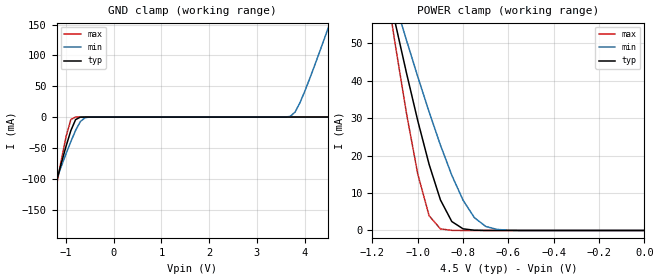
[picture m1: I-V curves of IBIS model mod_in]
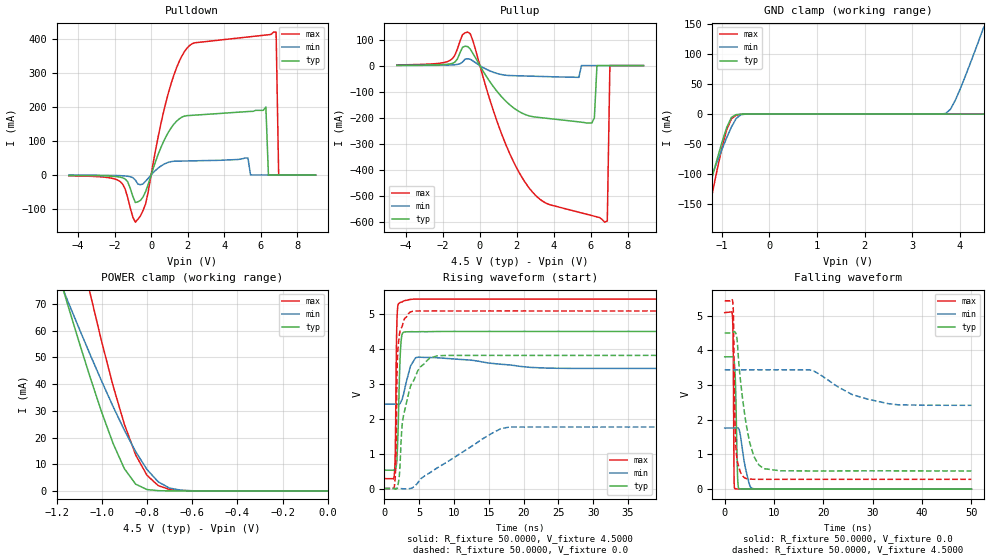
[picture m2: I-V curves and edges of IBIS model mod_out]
| IBIS file 54ac16244.ibs created by s2ibis3 verion 1.1
| North Carolina State University, ERL, 2006
[IBIS ver]  4.0
[File name] 54ac16244_4v5_rev1.ibs
[File Rev] 1.0
[Date]   19 Oct 2011
[Source] CAD & Design Solution (Catania) - STMicroelectronics
[Notes]
  (Note1) This IBIS model is the model of the product with package
   (Flat48 package elements);
  (Note2) This IBIS model is extracted with nominal 4.5V power supply
   (min:3.0V, typ:4.5V, max:5.5V);
  (Note3) This model has few Warnings about the non-monotonicity
   of I-V curves, but they are not indicative of problems
   inside the model;
[Copyright] (c) 2011 STMicroelectronics
|   Component 54AC16244
[Component] 54AC16244
[Manufacturer] STMicroelectronics
[Package]
| variable  typ   min   max
R_pkg   0.0   0.0   0.0
L_pkg   0.0H   0.0H   0.0H
C_pkg   0.0F   0.0F   0.0F
[Pin]  signal_name   model_name   R_pin   L_pin   C_pin
1   N1GN   mod_in   507.450m   7.328nH   1.49pF
2   N1Y1   mod_out   507.450m   7.328nH   1.49pF
3   N1Y2   mod_out   507.450m   7.328nH   1.49pF
4   GND1   GND   520.320m   7.732nH   1.49pF
5   N1Y3   mod_out   199.836m   3.681nH   1.24pF
6   N1Y4   mod_out   196.159m   3.561nH   1.24pF
7   VCC1   POWER   190.643m   3.384nH   1.24pF
8   N2Y1   mod_out   186.966m   3.268nH   1.24pF
9   N2Y2   mod_out   183.288m   3.154nH   1.24pF
10   GND2   GND   181.450m   3.098nH   1.24pF
11   N2Y3   mod_out   177.773m   2.987nH   1.24pF
12   N2Y4   mod_out   177.773m   2.987nH   1.24pF
13   N3Y1   mod_out   177.773m   2.987nH   1.24pF
14   N3Y2   mod_out   192.482m   3.443nH   1.24pF
15   GND3   GND   181.450m   3.098nH   1.24pF
16   N3Y3   mod_out   185.127m   3.211nH   1.24pF
17   N3Y4   mod_out   186.966m   3.268nH   1.24pF
18   VCC2   POWER   190.643m   3.384nH   1.24pF
19   N4Y1   mod_out   196.159m   3.561nH   1.24pF
20   N4Y2   mod_out   199.836m   3.681nH   1.24pF
21   GND4   GND   516.643m   7.614nH   1.49pF
22   N4Y3   mod_out   505.611m   7.272nH   1.49pF
23   N4Y4   mod_out   505.611m   7.272nH   1.49pF
24   N4GN   mod_in   505.611m   7.272nH   1.49pF
25   N3GN   mod_in   503.773m   7.217nH   1.49pF
26   N4A4   mod_in   503.773m   7.217nH   1.49pF
27   N4A3   mod_in   503.773m   7.217nH   1.49pF
28   GND5   GND   516.643m   7.614nH   1.49pF
29   N4A2   mod_in   201.675m   3.741nH   1.24pF
30   N4A1   mod_in   197.997m   3.621nH   1.24pF
31   VCC3   POWER   192.482m   3.443nH   1.24pF
32   N3A4   mod_in   186.966m   3.268nH   1.24pF
33   N3A3   mod_in   185.127m   3.211nH   1.24pF
34   GND6   GND   183.288m   3.154nH   1.24pF
35   N3A2   mod_in   181.450m   3.098nH   1.24pF
36   N3A1   mod_in   179.611m   3.042nH   1.24pF
37   N2A4   mod_in   179.611m   3.042nH   1.24pF
38   N2A3   mod_in   179.611m   3.042nH   1.24pF
39   GND7   GND   179.611m   3.042nH   1.24pF
40   N2A2   mod_in   185.127m   3.211nH   1.24pF
41   N2A1   mod_in   186.966m   3.268nH   1.24pF
42   VCC4   POWER   192.482m   3.443nH   1.24pF
43   N1A4   mod_in   196.159m   3.561nH   1.24pF
44   N1A3   mod_in   199.836m   3.681nH   1.24pF
45   GND8   GND   520.320m   7.732nH   1.49pF
46   N1A2   mod_in   509.288m   7.384nH   1.49pF
47   N1A1   mod_in   509.288m   7.384nH   1.49pF
48   N2GN   mod_in   505.611m   7.272nH   1.49pF
| Models and submodels in the file (2): mod_in (Input), mod_out (3-state)
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|   Model mod_in
[Model]   mod_in
Model_type Input
Vinl   =   1.3500V
Vinh   =   3.1500V
C_comp   0.5317pF   NA   NA
[Temperature Range]  25.0000   0.1250k   -55.0000
[Voltage Range]   4.5000V   3.0000V   5.5000V
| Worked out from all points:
|   GND clamp passes 1 mA (typ) near -0.72 V on its own axis
|   POWER clamp passes 1 mA (typ) near -0.81 V on its own axis
[GND_clamp]
|Voltage   I(typ)   I(min)   I(max)
-4.5V     -1.124A    -840.2mA   -1.572A
-1.7V     -254mA     -209.8mA   -326.6mA
-1.6V     -223.6mA   -187.8mA   -282.8mA
-1.5V     -193.3mA   -165.8mA   -239.3mA
-1.4V     -163.2mA   -144mA     -196mA
-1V       -47.28mA   -59.41mA   -31.62mA
-900mV    -22mA      -39.68mA   -4.062mA
-800mV    -4.121mA   -21.58mA   -32.26uA
-500mV    -58.62nA   -53.9uA    -16.8pA
3.7V      5.8pA      1.071mA    3.8pA
3.9V      6.6pA      22.78mA    4.6pA
4.5V      9pA        145.6mA    7pA
[POWER_clamp]
|Voltage   I(typ)   I(min)   I(max)
-4.5V     1.102A     819.1mA    1.549A
-1.15V    69.48mA    71.07mA    69.5mA
-1.1V     55.56mA    60.84mA    49.84mA
-1.05V    42.07mA    50.81mA    31.3mA
-1V       29.27mA    41.04mA    15.03mA
-950mV    17.64mA    31.64mA    3.932mA
-900mV    8.156mA    22.78mA    419.2uA
-850mV    2.388mA    14.75mA    30.75uA
-800mV    435.6uA    8.064mA    2.159uA
-750mV    65.2uA     3.407mA    151.1nA
-700mV    9.379uA    1.071mA    10.58nA
0V        9pA        45.39pA    11pA
|   Model mod_out
[Model]   mod_out
Model_type 3-state
Enable   Active-Low
Vmeas  =   2.25V
Cref   =   50pF
Rref   =   500
C_comp   1.464pF   NA   NA
[Temperature Range]   25.0000   0.1250k   -55.0000
[Voltage Range]   4.5000V   3.0000V   5.5000V
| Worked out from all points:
|   slope of the pulldown table from 0 to 0.675 V, typ, clamps not added: 6.92 ohm
|   slope of the pullup table from 0 to 0.675 V, typ, clamps not added: 8.98 ohm
|   GND clamp passes 1 mA (typ) near -0.70 V on its own axis
|   POWER clamp passes 1 mA (typ) near -0.81 V on its own axis
|   rising waveform, R_fixture 50.0000, V_fixture 4.5000: 20-80 % time 350ps typ, 745ps min, 173ps max; typ from 0.527 V to 4.5 V
|   rising waveform, R_fixture 50.0000, V_fixture 0.0: 20-80 % time 1.81ns typ, 8.3ns min, 312ps max; typ from 0 V to 3.81 V
|   falling waveform, R_fixture 50.0000, V_fixture 0.0: 20-80 % time 354ps typ, 1.29ns min, 133ps max; typ from 3.81 V to 0 V
|   falling waveform, R_fixture 50.0000, V_fixture 4.5000: 20-80 % time 2.29ns typ, 8.32ns min, 397ps max; typ from 4.5 V to 0.526 V
[Pulldown]
|Voltage   I(typ)   I(min)   I(max)
-4.5V     -1.2mA     -500uA     -2.4mA
-1.7V     -6.41mA    -2.03mA    -19.12mA
-860mV    -81.02mA   -14.97mA   -138.8mA
-300mV    -48.8mA    -18.04mA   -84.82mA
1.1V      138.7mA    39.35mA    269.5mA
1.94V     174.3mA    41.15mA    371.1mA
6.28V     200mA      0A         411.4mA
6.42V     0A         0A         412.2mA
6.7V      0A         0A         420mA
6.84V     0A         0A         420mA
6.98V     0A         0A         0A
9V        0A         0A         0A
[Pullup]
|Voltage   I(typ)   I(min)   I(max)
-4.5V     1mA        460uA      2.7mA
-1.64V    6.19mA     2.12mA     18.86mA
-520mV    63.45mA    24.32mA    121.8mA
1.16V     -118.1mA   -34.17mA   -258.5mA
2.56V     -190.3mA   -40.04mA   -458.5mA
6.06V     -220mA     0A         -574.6mA
6.2V      -200mA     0A         -577.2mA
6.34V     0A         0A         -579.7mA
6.76V     0A         0A         -600mA
6.9V      0A         0A         -595mA
7.04V     0A         0A         0A
8.86V     0A         0A         0A
[GND_clamp]
|Voltage   I(typ)   I(min)   I(max)
-4.5V     -1.124A    -840.2mA   -1.58A
-1.7V     -254.2mA   -209.8mA   -342.2mA
-1.6V     -223.7mA   -187.8mA   -299.2mA
-1.5V     -193.4mA   -165.9mA   -256.6mA
-1.4V     -163.4mA   -144.1mA   -214.5mA
-1.3V     -133.5mA   -122.5mA   -173mA
-900mV    -22.73mA   -39.76mA   -26.64mA
-700mV    -857.1uA   -7.393mA   -1.921mA
-500mV    -11.95uA   -74.71uA   -9.782uA
3.7V      83.63pA    1.058mA    9.733pA
3.9V      87.56pA    22.74mA    11.74pA
4.5V      103.8pA    145.6mA    17.76pA
[POWER_clamp]
|Voltage   I(typ)   I(min)   I(max)
-4.5V     1.102A     819.1mA    1.573A
-1.2V     83.8mA     81.43mA    130.9mA
-1.15V    69.58mA    71.05mA    111.2mA
-1.05V    42.19mA    50.78mA    73.46mA
-950mV    17.8mA     31.61mA    39.39mA
-900mV    8.328mA    22.74mA    24.97mA
-850mV    2.531mA    14.72mA    13.47mA
-800mV    511.9uA    8.027mA    5.851mA
-750mV    95.36uA    3.379mA    1.971mA
-700mV    20.21uA    1.058mA    551.7uA
-650mV    5.117uA    272.8uA    145.4uA
0V        103.8pA    0A         31.8pA
[Ramp]
| variable   typ   min   max
dV/dt_r  2.2882/1.8552n   1.0568/12.4296n   3.0522/0.3861n
dV/dt_f  2.3844/2.2782n   1.1656/14.8921n   3.0888/0.7097n
R_load = 50.0000
[Rising Waveform]
R_fixture= 50.0000
V_fixture= 4.5000
|time   V(typ)   V(min)   V(max)
0s        526.6mV    2.416V     283.7mV
1.4ns     528.5mV    2.416V     340.8mV
1.55ns    545.6mV    2.415V     975.8mV
1.7ns     647.8mV    2.414V     3.802V
1.8ns     820.3mV    2.413V     4.827V
2.25ns    3.723V     2.441V     5.329V
2.6ns     4.449V     2.594V     5.352V
3.75ns    4.493V     3.509V     5.418V
4.85ns    4.492V     3.763V     5.428V
50ns      4.5V       3.44V      5.428V
[Rising Waveform]
R_fixture= 50.0000
V_fixture= 0.0
|time   V(typ)   V(min)   V(max)
0s        140.5pV    0V         93.97pV
1.4ns     -1.409mV   -18.99uV   17.29mV
1.6ns     -16.83mV   -12.64uV   518.1mV
1.8ns     12.24mV    159.2uV    3.217V
2ns       156.2mV    580.3uV    4.135V
2.6ns     1.922V     -5.928mV   4.685V
3.7ns     2.896V     -777uV     5.055V
6.5ns     3.735V     448.3mV    5.087V
17.95ns   3.814V     1.762V     5.087V
50ns      3.814V     1.761V     5.087V
[Falling Waveform]
R_fixture= 50.0000
V_fixture= 0.0
|time   V(typ)   V(min)   V(max)
0s        3.814V     1.762V     5.087V
1.6ns     3.816V     1.761V     4.923V
1.75ns    3.815V     1.761V     3.614V
1.9ns     3.707V     1.761V     265.6mV
2.05ns    3.466V     1.762V     18.58mV
2.25ns    2.701V     1.764V     8.995mV
2.6ns     406.5mV    1.767V     4.599mV
2.9ns     15.44mV    1.722V     5.676mV
5.65ns    2.208mV    19.14mV    254.8uV
50ns      -22.61uV   4.808uV    31.83uV
[Falling Waveform]
R_fixture= 50.0000
V_fixture= 4.5000
|time   V(typ)   V(min)   V(max)
0s        4.5V       3.44V      5.428V
1.65ns    4.508V     3.44V      5.373V
1.8ns     4.537V     3.44V      4.806V
2.05ns    4.536V     3.44V      2.15V
2.25ns    4.489V     3.44V      1.241V
3.9ns     2.316V     3.44V      338.5mV
5.9ns     951.2mV    3.44V      285.1mV
7.9ns     591.7mV    3.44V      283.8mV
33.15ns   527.1mV    2.464V     283.6mV
50ns      525.9mV    2.416V     283.8mV
